(* Logix 5000 AddOnInstructionDefinition export Banner_R95_8B22_R130C_PD_v4; software revision 33.00 *)

TYPE Banner_R95C_R130C_8B22_PD_v4 :   // UDT that records the converted prcoess data.
STRUCT
   DTI : SINT[2];   // Data Transfer In
   DTO : SINT[2];   // Data Transfer Out
   Port_Data : Banner_R95C_R130C_8B22_Port_Data_v4[9];
END_STRUCT
END_TYPE

TYPE Banner_R95C_R130C_8B22_Port_Data_v4 :
STRUCT
   Discrete_1_In : BOOL;
   Discrete_2_In : BOOL;
   Discrete_1_Out : BOOL;
   Discrete_2_Out : BOOL;
END_STRUCT
END_TYPE

ADD_ON_INSTRUCTION Banner_R95_8B22_R130C_PD_v4   (* revision 4.0, vendor Banner Engineering *)
// Takes the raw SINT information and converts that data into actual information.
VAR_IN_OUT
   PD : Banner_R95C_R130C_8B22_PD_v4; {required}
END_VAR
VAR_INPUT
   Byte_Swap : BOOL; {required}   // Swap the LSB and the MSB with each other.
END_VAR
VAR
   Temp_Measurement : DINT; {access None}
   Byte_Out : SINT[2]; {access None}
   Byte_In : SINT[2]; {access None}
END_VAR

ROUTINE Logic   (* ladder *)
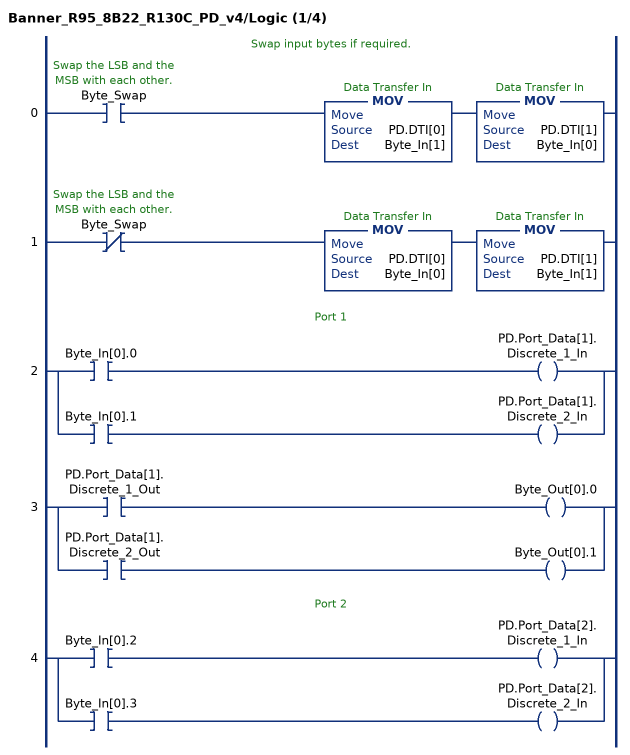
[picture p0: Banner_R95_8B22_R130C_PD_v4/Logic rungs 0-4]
   // Swap input bytes if required.
   0: XIC(Byte_Swap)MOV(PD.DTI[0],Byte_In[1])MOV(PD.DTI[1],Byte_In[0]);
   1: XIO(Byte_Swap)MOV(PD.DTI[0],Byte_In[0])MOV(PD.DTI[1],Byte_In[1]);
   // Port 1
   2: [XIC(Byte_In[0].0) OTE(PD.Port_Data[1].Discrete_1_In) ,XIC(Byte_In[0].1) OTE(PD.Port_Data[1].Discrete_2_In) ];
   3: [XIC(PD.Port_Data[1].Discrete_1_Out) OTE(Byte_Out[0].0) ,XIC(PD.Port_Data[1].Discrete_2_Out) OTE(Byte_Out[0].1) ];
   // Port 2
   4: [XIC(Byte_In[0].2) OTE(PD.Port_Data[2].Discrete_1_In) ,XIC(Byte_In[0].3) OTE(PD.Port_Data[2].Discrete_2_In) ];
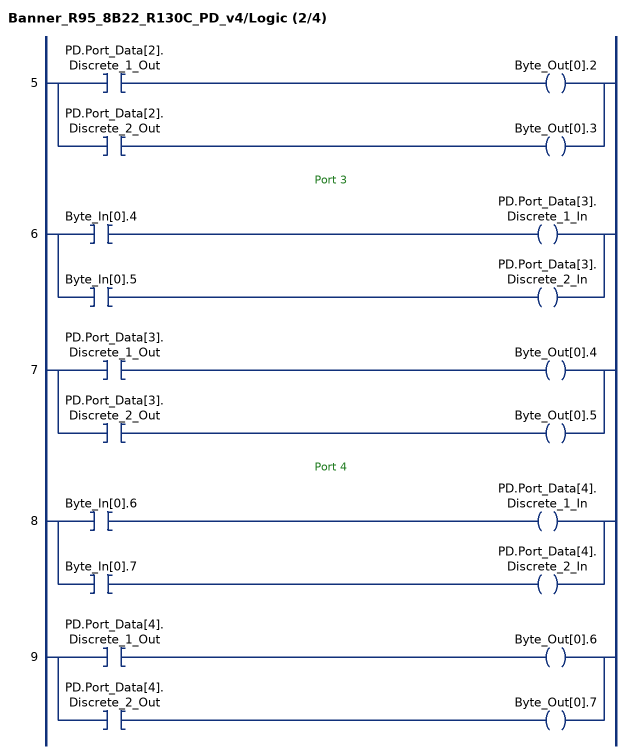
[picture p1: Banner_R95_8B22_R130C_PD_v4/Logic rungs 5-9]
   5: [XIC(PD.Port_Data[2].Discrete_1_Out) OTE(Byte_Out[0].2) ,XIC(PD.Port_Data[2].Discrete_2_Out) OTE(Byte_Out[0].3) ];
   // Port 3
   6: [XIC(Byte_In[0].4) OTE(PD.Port_Data[3].Discrete_1_In) ,XIC(Byte_In[0].5) OTE(PD.Port_Data[3].Discrete_2_In) ];
   7: [XIC(PD.Port_Data[3].Discrete_1_Out) OTE(Byte_Out[0].4) ,XIC(PD.Port_Data[3].Discrete_2_Out) OTE(Byte_Out[0].5) ];
   // Port 4
   8: [XIC(Byte_In[0].6) OTE(PD.Port_Data[4].Discrete_1_In) ,XIC(Byte_In[0].7) OTE(PD.Port_Data[4].Discrete_2_In) ];
   9: [XIC(PD.Port_Data[4].Discrete_1_Out) OTE(Byte_Out[0].6) ,XIC(PD.Port_Data[4].Discrete_2_Out) OTE(Byte_Out[0].7) ];
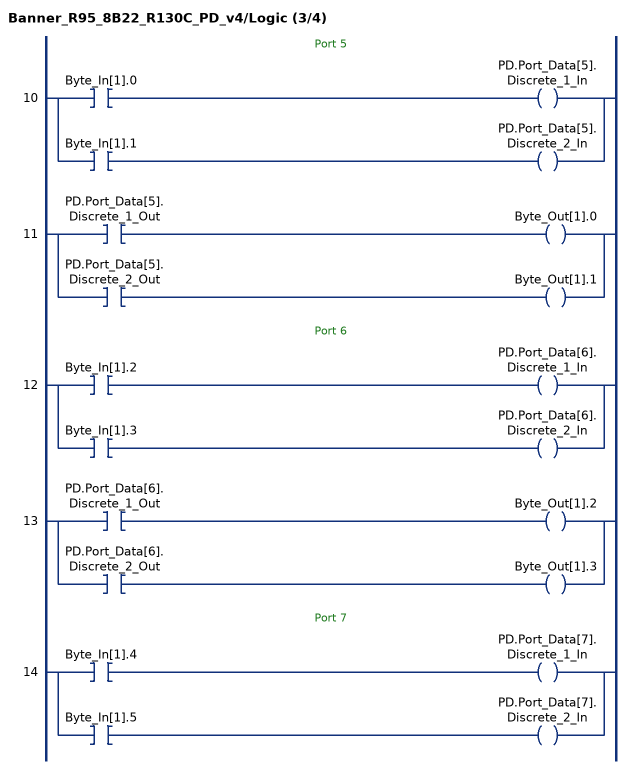
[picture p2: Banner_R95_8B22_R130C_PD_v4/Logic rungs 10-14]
   // Port 5
   10: [XIC(Byte_In[1].0) OTE(PD.Port_Data[5].Discrete_1_In) ,XIC(Byte_In[1].1) OTE(PD.Port_Data[5].Discrete_2_In) ];
   11: [XIC(PD.Port_Data[5].Discrete_1_Out) OTE(Byte_Out[1].0) ,XIC(PD.Port_Data[5].Discrete_2_Out) OTE(Byte_Out[1].1) ];
   // Port 6
   12: [XIC(Byte_In[1].2) OTE(PD.Port_Data[6].Discrete_1_In) ,XIC(Byte_In[1].3) OTE(PD.Port_Data[6].Discrete_2_In) ];
   13: [XIC(PD.Port_Data[6].Discrete_1_Out) OTE(Byte_Out[1].2) ,XIC(PD.Port_Data[6].Discrete_2_Out) OTE(Byte_Out[1].3) ];
   // Port 7
   14: [XIC(Byte_In[1].4) OTE(PD.Port_Data[7].Discrete_1_In) ,XIC(Byte_In[1].5) OTE(PD.Port_Data[7].Discrete_2_In) ];
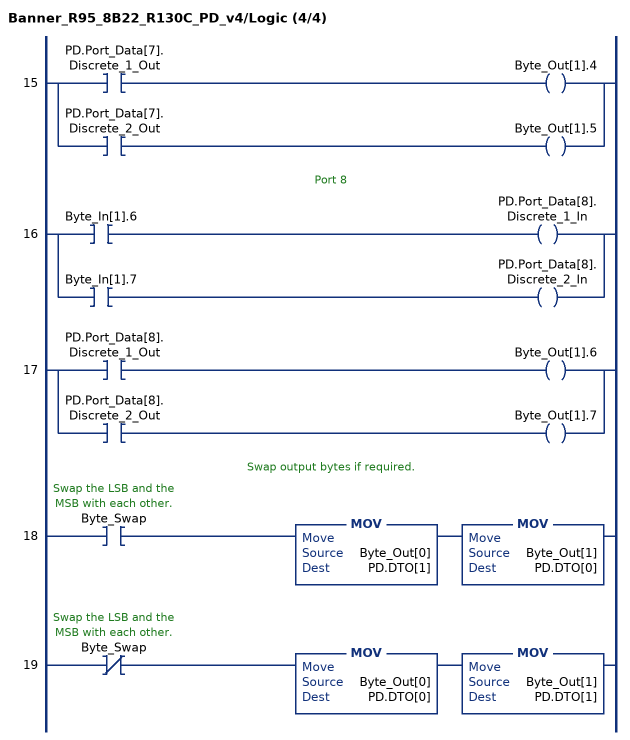
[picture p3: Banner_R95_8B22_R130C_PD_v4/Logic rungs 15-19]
   15: [XIC(PD.Port_Data[7].Discrete_1_Out) OTE(Byte_Out[1].4) ,XIC(PD.Port_Data[7].Discrete_2_Out) OTE(Byte_Out[1].5) ];
   // Port 8
   16: [XIC(Byte_In[1].6) OTE(PD.Port_Data[8].Discrete_1_In) ,XIC(Byte_In[1].7) OTE(PD.Port_Data[8].Discrete_2_In) ];
   17: [XIC(PD.Port_Data[8].Discrete_1_Out) OTE(Byte_Out[1].6) ,XIC(PD.Port_Data[8].Discrete_2_Out) OTE(Byte_Out[1].7) ];
   // Swap output bytes if required.
   18: XIC(Byte_Swap)MOV(Byte_Out[0],PD.DTO[1])MOV(Byte_Out[1],PD.DTO[0]);
   19: XIO(Byte_Swap)MOV(Byte_Out[0],PD.DTO[0])MOV(Byte_Out[1],PD.DTO[1]);
END_ROUTINE
END_ADD_ON_INSTRUCTION
